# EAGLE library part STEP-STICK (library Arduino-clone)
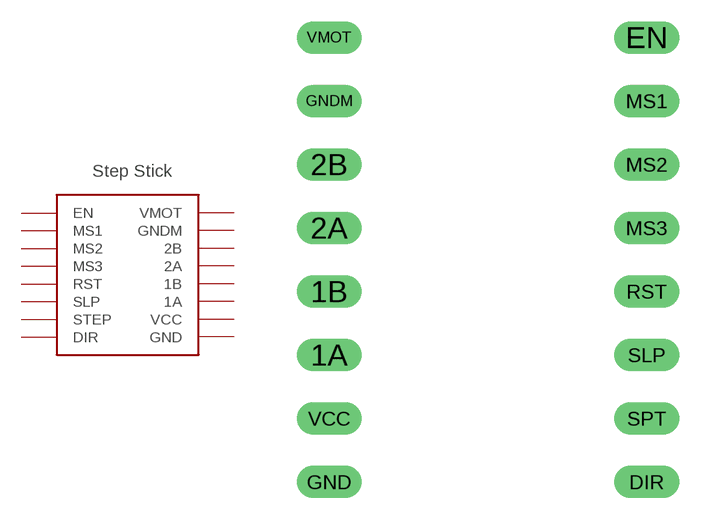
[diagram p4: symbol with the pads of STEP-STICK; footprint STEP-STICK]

Designator prefix -

## STEP-STICK  [STEP-STICK]
1A  1A
1B  1B
2A  2A
2B  2B
DIR  DIR
EN  EN
GND  GND
GNDM  GNDM
MS1  MS1
MS2  MS2
MS3  MS3
RST  RST
SLP  SLP
SPT  STEP
VCC  VCC
VMOT  VMOT

## Footprint STEP-STICK (pad centres in mm)
drill 0.8 long: 1A -8.89,-7.62; 1B -8.89,-5.08; 2A -8.89,-2.54; 2B -8.89,0; DIR 3.81,-12.7; EN 3.81,5.08; GND -8.89,-12.7; GNDM -8.89,2.54; MS1 3.81,2.54; MS2 3.81,0; MS3 3.81,-2.54; RST 3.81,-5.08; SLP 3.81,-7.62; SPT 3.81,-10.16; VCC -8.89,-10.16; VMOT -8.89,5.08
